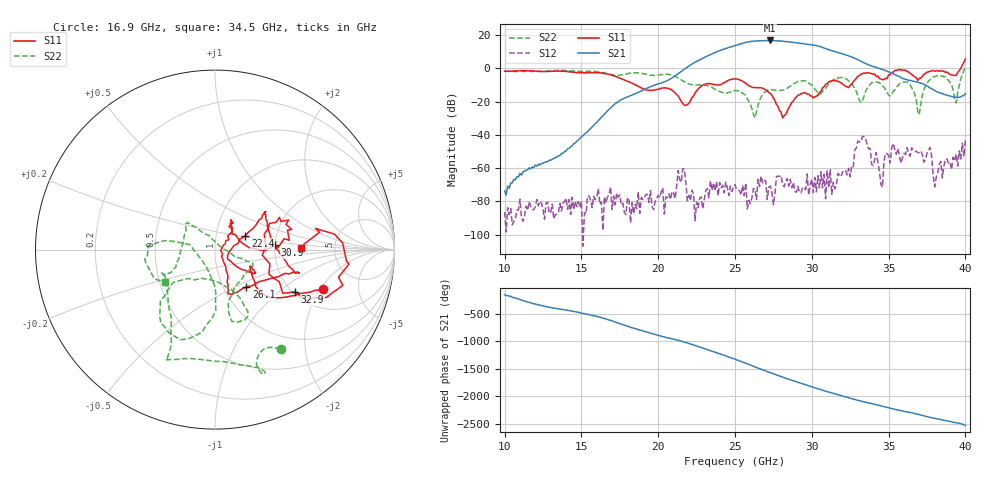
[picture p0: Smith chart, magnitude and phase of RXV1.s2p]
!Keysight Technologies,M9808A,MY58100618,A.14.70.03
!Date: Monday, February 27, 2023 13:43:48
!Correction: S11(Cdelta 2-Port  )
!S21(Cdelta 2-Port  )
!S12(Cdelta 2-Port  )
!S22(Cdelta 2-Port  )
!S2P File: Measurements: S11, S21, S12, S22:
# Hz S  RI  R 50
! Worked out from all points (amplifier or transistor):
!   301 points, 10 GHz to 40 GHz, reference 50 ohm
!   highest |S21| = 16.9 dB at 27.3 GHz (marker M1)
!   |S21| within 3 dB of that: 25.02 GHz to 30.25 GHz (5.23 GHz wide, 18.9 % of centre)
!   unconditionally stable (mu >= 1): start of sweep to 39.64 GHz
!   at 15 GHz: K = 83809.31, MAG = -33.0 dB, |S12| = -79.8 dB
!   at 25 GHz: K = 232.87, MAG = 15.1 dB, |S12| = -69.9 dB
!   at 40 GHz: K = 385.29, MSG = 14.0 dB, |S12| = -43.1 dB
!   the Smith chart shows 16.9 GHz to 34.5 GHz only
!   S11 on the Smith chart (normalised r, x): 16.9 GHz: 2.86, -2.14; 22.4 GHz: 1.39, +0.22; 26.1 GHz: 1.28, -0.57; 30.9 GHz: 2.00, +0.11; 32.9 GHz: 2.05, -1.29; 34.5 GHz: 2.86, +0.07
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1e10  0.1026 0.8219  -0.000182 -9.83e-05  -4.44e-05 -1.78e-05  0.6887 0.4623
1.5e10  0.7343 0.0718  -0.00499 -0.00698  9.58e-05 3.46e-05  0.6586 -0.4949
1.69e10  0.6036 -0.2201  -0.00953 0.0645  0.000164 0.00022  0.365 -0.5512
2e10  0.2091 -0.1096  -0.3419 -0.0353  -0.000133 -7.34e-05  -0.1789 -0.6079
2.24e10  0.1686 0.0757  1.539 0.1017  7.85e-06 -2.49e-05  -0.287 -0.1358
2.38e10  0.2922 0.1243  -1.884 -2.508  -0.000311 0.000231  -0.2167 -0.0742
2.44e10  0.3956 -0.0658  -3.967 0.4053  -5.67e-05 0.000373  -0.1717 0.0514
2.5e10  0.4657 -0.1277  -2.013 4.454  8.52e-05 -0.000309  -0.1631 0.1454
2.56e10  0.3548 -0.15  3.579 4.689  -2.41e-05 -0.000146  -0.1096 0.128
2.61e10  0.1749 -0.2075  6.557 -0.3134  4.04e-05 0.000119  -0.0178 0.0592
2.67e10  0.0821 -0.2489  2.517 -6.37  0.000332 -0.000477  0.1281 -0.0454
2.73e10  0.072 -0.159  -4.539 -5.278  0.000265 0.000121  0.2115 -0.0841
2.79e10  0.0364 -0.0389  -6.614 1.435  -8.34e-05 0.000562  0.161 -0.145
2.86e10  0.0598 0.0493  -1.166 6.133  0.000108 0.000453  0.0779 -0.2804
2.93e10  0.0936 0.1483  4.504 3.456  -0.000172 -4.84e-05  0.1437 -0.3987
3e10  0.0924 0.1172  4.644 -2.17  0.000317 -0.000341  0.1471 -0.2798
3.09e10  0.3336 0.0248  -1.102 -3.847  -0.000111 -4.63e-05  -0.1858 -0.1698
3.17e10  0.3666 0.157  -2.974 -0.5481  0.000413 0.000562  -0.2789 -0.4325
3.29e10  0.4445 -0.2356  -0.2051 1.91  -0.000754 -0.00397  -0.00185 -0.2023
3.45e10  0.4818 0.00962  0.9427 -0.1921  -0.00022 0.000239  -0.2758 -0.1798
3.5e10  0.5413 -0.3496  0.5445 -0.583  0.00237 0.000559  0.0028 -0.1587
4e10  0.8849 -1.704  0.1736 -0.0246  0.00667 0.00217  0.5919 -1
